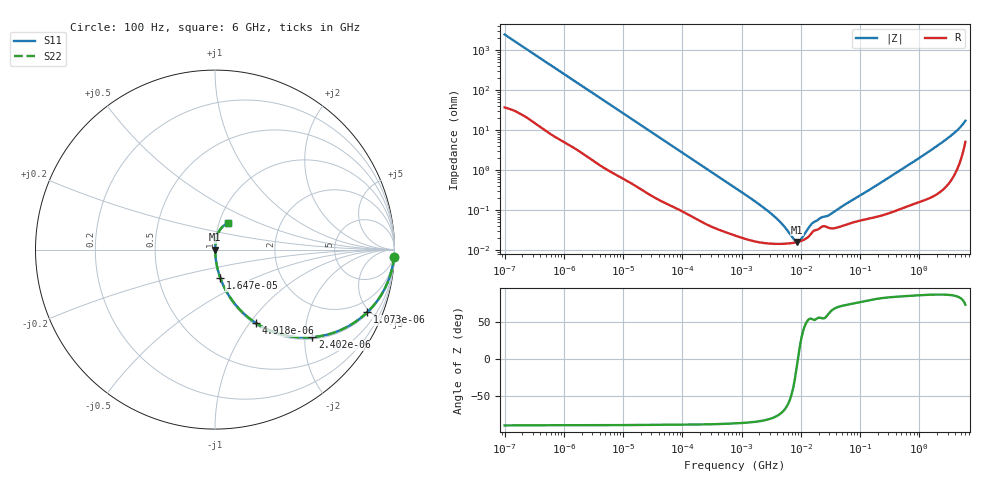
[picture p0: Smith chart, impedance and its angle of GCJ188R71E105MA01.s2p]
!Murata Part Number: GCJ188R71E105MA01
!These Parameters are Measured in Series Mode Connection
!Data Generated on Mar 13, 2026
!  o--ll--o
!Port1  Port2
!  o------o
!Operation Temp=25[degC], DC Bias Voltage=0[V]
!Freq. Start=100[Hz] Stop=6[GHz] 401[Steps]
# Hz S RI R 50
!Freq.(Hz) S11(Real) S11(Imag) S21(Real) S21(Imag) S12(Real) S12(Imag) S22(Real) S22(Imag)
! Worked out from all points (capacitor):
!   401 points, 100 Hz to 6 GHz, reference 50 ohm
!   read as one part in series: C = 632 nF near 109 Hz
!   lowest |Z| = 16.2 mohm at 8.692 MHz (marker M1)
!   series resonance near 8.938 MHz, so ESL is about 500 pH
!   S11 on the Smith chart (normalised r, x): 100 Hz: 2, -50; 1.073 kHz: 1.10, -4.82; 2.402 kHz: 1.05, -2.18; 4.918 kHz: 1.02, -1.07; 16.47 kHz: 1.01, -0.33; 6 GHz: 1.10, +0.33
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100  0.9978 -0.0398  0.00218 0.0398  0.00218 0.0398  0.9978 -0.0398
366  0.9773 -0.1397  0.0227 0.1397  0.0227 0.1397  0.9773 -0.1397
656  0.935 -0.2373  0.065 0.2373  0.065 0.2373  0.935 -0.2373
1073  0.8482 -0.349  0.1518 0.349  0.1518 0.349  0.8482 -0.349
2008  0.6254 -0.4736  0.3746 0.4736  0.3746 0.4736  0.6254 -0.4736
2402  0.5416 -0.4879  0.4584 0.4879  0.4584 0.4879  0.5416 -0.4879
4918  0.2283 -0.4094  0.7717 0.4094  0.7717 0.4094  0.2283 -0.4094
8416  0.0958 -0.2833  0.9042 0.2833  0.9042 0.2833  0.0958 -0.2833
16473  0.0296 -0.1575  0.9704 0.1575  0.9704 0.1575  0.0296 -0.1575
40335  0.00632 -0.0669  0.9937 0.0669  0.9937 0.0669  0.00632 -0.0669
774597  0.000248 -0.00369  0.9998 0.00369  0.9998 0.00369  0.000248 -0.00369
3394479  0.000147 -0.000742  0.9999 0.000742  0.9999 0.000742  0.000147 -0.000742
5079039  0.000146 -0.000394  0.9999 0.000394  0.9999 0.000394  0.000146 -0.000394
7599586  0.000154 -0.000108  0.9998 0.000108  0.9998 0.000108  0.000154 -0.000108
8692127  0.000161 -1.85e-05  0.9998 1.85e-05  0.9998 1.85e-05  0.000161 -1.85e-05
9941735  0.00017 7.2e-05  0.9998 -7.2e-05  0.9998 -7.2e-05  0.00017 7.2e-05
1.555665e7  0.000283 0.000382  0.9997 -0.000382  0.9997 -0.000382  0.000283 0.000382
2.225763e7  0.000383 0.000544  0.9996 -0.000544  0.9996 -0.000544  0.000383 0.000544
3.045065e7  0.000362 0.000681  0.9996 -0.000681  0.9996 -0.000681  0.000362 0.000681
3.124326e8  0.000898 0.00668  0.9991 -0.00668  0.9991 -0.00668  0.000898 0.00668
2.450438e9  0.00571 0.0502  0.9943 -0.0502  0.9943 -0.0502  0.00571 0.0502
6e9  0.0726 0.1473  0.9274 -0.1473  0.9274 -0.1473  0.0726 0.1473
